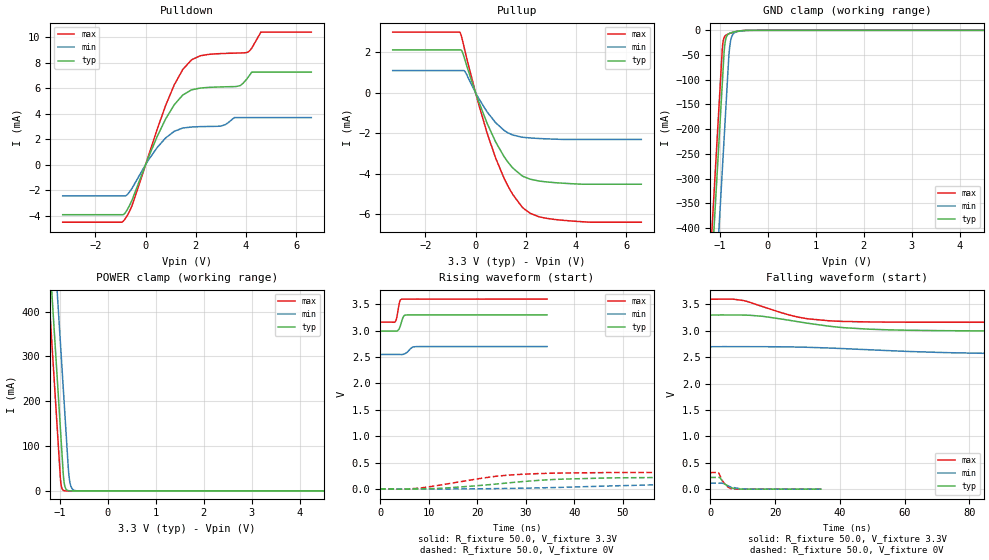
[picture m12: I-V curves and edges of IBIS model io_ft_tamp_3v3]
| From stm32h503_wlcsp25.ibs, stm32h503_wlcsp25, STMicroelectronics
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[Model]   io_ft_tamp_3v3
Model_type I/O
Polarity   Non-Inverting
Enable   Active-Low
| CAP_THRESHOLD on pad IOFT is "UDTCAPC" :
| Rising=20.0% of vddios   Falling=80.0% of vddios
| C_comp min and max val. don't necessarily correlate with the min and max pvt
| but are the smallest and greatest pad capacitance found.
| var   typ   min   max
C_comp   2.63002pF  2.62265pF  2.64550pF
|C_comp_pullup   1.52890pF  1.47780pF  1.43435pF
|C_comp_pulldown   1.10112pF  1.14485pF  1.21115pF
Vinl = 810.0mV
Vinh = 2.52V
Vmeas = 1.65V   | Reference voltage for timing measurements
Cref  = 50.0pF   | Timing specification test load capacitance value
Rref  = 100.0MOhm   | Timing specification test load resistance value
Vref  = 1.65V   | Timing specification test load voltage
[Model Spec]
| TIME_THRESHOLD on pin ZIV11 is "CMOS" :
| Rising=40.0% of vdd   Falling=60.0% of vdd
Vinl 1.29880V 1.07480V 1.40680V
Vinh 1.77520V 1.49320V 1.89720V
| variable   typ   min   max
[Temperature Range] 25.0 125.0 -40.0
| variable   typ   min   max
[Voltage Range] 3.3V 2.7V 3.6V
| variable   typ   min   max
[POWER Clamp Reference] 3.3V 2.7V 3.6V
| variable   typ   min   max
[GND Clamp Reference] 0V 0V 0V
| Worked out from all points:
|   slope of the pulldown table from 0 to 0.495 V, typ, clamps not added: 211 ohm
|   slope of the pullup table from 0 to 0.495 V, typ, clamps not added: 307 ohm
|   GND clamp passes 1 mA (typ) near -0.57 V on its own axis
|   POWER clamp passes 1 mA (typ) near -0.84 V on its own axis
|   rising waveform, R_fixture 50.0, V_fixture 3.3V: 20-80 % time 642ps typ, 1.02ns min, 501ps max; typ from 2.99 V to 3.3 V
|   falling waveform, R_fixture 50.0, V_fixture 3.3V: 20-80 % time 22.1ns typ, 40.9ns min, 14.5ns max; typ from 3.3 V to 2.99 V
|   rising waveform, R_fixture 50.0, V_fixture 0V: 20-80 % time 17.9ns typ, 30.6ns min, 13.4ns max; typ from 0 V to 0.222 V
|   falling waveform, R_fixture 50.0, V_fixture 0V: 20-80 % time 2.43ns typ, 3.42ns min, 2.02ns max; typ from 0.222 V to 0 V
[POWER Clamp]
-3.3V     4.068A     4.259A     3.957A
-1.24V    565.8mA    757.2mA    454.5mA
-1.17V    446.8mA    638.2mA    335.5mA
-1.13V    378.8mA    570.2mA    267.5mA
-1.05V    242.8mA    434.2mA    131.5mA
-980mV    123.8mA    315.2mA    17.95mA
-920mV    26.3mA     213.2mA    906uA
-880mV    5.543mA    145.2mA    123.7uA
-810mV    363.5uA    33.6mA     3.797uA
-770mV    76.62uA    10.47mA    518.9nA
-690mV    3.404uA    1.017mA    9.9nA
6.6V      0A         0A         0A
[GND Clamp]
-3.3V     -4.103A    -4.279A    -4.033A
-1.25V    -618.3mA   -794.4mA   -547.9mA
-960mV    -125.3mA   -301.4mA   -54.9mA
-950mV    -108.3mA   -284.4mA   -38.2mA
-930mV    -74.28mA   -250.4mA   -21.25mA
-910mV    -41.9mA    -216.3mA   -14.37mA
-890mV    -23.93mA   -182.3mA   -11.25mA
-810mV    -6.829mA   -48.78mA   -6.737mA
-780mV    -5.411mA   -23.28mA   -5.701mA
-690mV    -2.92mA    -4.615mA   -3.19mA
-410mV    -72.95uA   -208.4uA   -32.16uA
6.6V      3.146nA    586.1nA    192.6pA
| variable   typ   min   max
[Pullup Reference] 3.3V 2.7V 3.6V
| variable   typ   min   max
[Pulldown Reference] 0V 0V 0V
[Pullup]
-3.3V     2.118mA    1.099mA    3.002mA
-620mV    2.118mA    1.099mA    2.981mA
-540mV    2.047mA    1.099mA    2.683mA
-420mV    1.614mA    1.045mA    2.057mA
120mV     -423.9uA   -273uA     -554.9uA
460mV     -1.518mA   -952.3uA   -2.004mA
800mV     -2.438mA   -1.486mA   -3.239mA
1.29V     -3.439mA   -1.987mA   -4.622mA
1.92V     -4.158mA   -2.21mA    -5.737mA
2.51V     -4.367mA   -2.265mA   -6.134mA
3.19V     -4.454mA   -2.3mA     -6.279mA
6.6V      -4.528mA   -2.313mA   -6.409mA
[Pulldown]
-3.3V     -3.931mA   -2.458mA   -4.52mA
-860mV    -3.894mA   -2.458mA   -4.374mA
-520mV    -2.688mA   -1.793mA   -3.111mA
800mV     3.6mA      2.103mA    4.66mA
1.48V     5.472mA    2.879mA    7.48mA
1.83V     5.88mA     2.962mA    8.24mA
2.99V     6.111mA    3.029mA    8.73mA
3.6V      6.141mA    3.701mA    8.772mA
4.05V     6.784mA    3.701mA    8.828mA
4.23V     7.274mA    3.701mA    9.167mA
4.59V     7.274mA    3.701mA    10.42mA
6.6V      7.274mA    3.701mA    10.42mA
[Ramp]
dV/dt_r 133.32371mV/17.75827ns 68.10059mV/30.01872ns 188.78366mV/13.44463ns
dV/dt_f 183.37683mV/21.75902ns 90.19237mV/40.12235ns 262.38588mV/14.4263ns
R_load = 50.0
| Removed startup time: 0s 0s 0s  .
| Removed end time: 34.4ns.
[Rising Waveform]
R_fixture   = 50.0
V_fixture   = 3.3V
V_fixture_min = 2.7V
V_fixture_max = 3.6V
0s        2.994V     2.55V      3.163V
3.05ns    2.994V     2.55V      3.168V
3.4ns     2.994V     2.55V      3.249V
4ns       3.057V     2.55V      3.55V
4.45ns    3.188V     2.549V     3.597V
4.75ns    3.263V     2.553V     3.599V
5.05ns    3.293V     2.564V     3.599V
6.5ns     3.3V       2.679V     3.599V
7.05ns    3.3V       2.696V     3.6V
34.4ns    3.3V       2.7V       3.6V
| Removed startup time: 0s 0s 0s  .
| Removed end time: 599.4ns.
[Falling Waveform]
R_fixture   = 50.0
V_fixture   = 3.3V
V_fixture_min = 2.7V
V_fixture_max = 3.6V
0s        3.3V       2.7V       3.6V
10.15ns   3.299V     2.7V       3.575V
16.3ns    3.275V     2.7V       3.456V
23.9ns    3.205V     2.696V     3.309V
30.2ns    3.143V     2.688V     3.227V
39.15ns   3.071V     2.669V     3.183V
48.95ns   3.032V     2.642V     3.169V
85.65ns   2.999V     2.573V     3.163V
134.6ns   2.995V     2.555V     3.163V
599.4ns   2.994V     2.55V      3.163V
| Removed startup time: 0s 0s 0s  .
| Removed end time: 599.4ns.
[Rising Waveform]
R_fixture   = 50.0
V_fixture   = 0V
V_fixture_min = 0V
V_fixture_max = 0V
0s        67.41nV    382.4nV    77.77nV
4.2ns     -2.094mV   -30.79uV   -2.95mV
8.1ns     1.219mV    -286.8uV   16.16mV
21.2ns    71.93mV    4.878mV    208.3mV
27ns      121mV      11.8mV     266.8mV
35.6ns    179.6mV    27.28mV    299.9mV
46.9ns    209.6mV    56.18mV    311.4mV
73.4ns    221.4mV    101.4mV    314.5mV
110.1ns   222.1mV    112.3mV    314.6mV
599.4ns   222.2mV    113.5mV    314.6mV
| Removed startup time: 0s 0s 0s  .
| Removed end time: 34.4ns.
[Falling Waveform]
R_fixture   = 50.0
V_fixture   = 0V
V_fixture_min = 0V
V_fixture_max = 0V
0s        222.2mV    113.5mV    314.6mV
2.5ns     222mV      113.5mV    314.3mV
3ns       216.3mV    113.5mV    255.8mV
3.65ns    162.5mV    114.5mV    167.2mV
4.45ns    99.12mV    93.46mV    102.5mV
5.7ns     51.26mV    56.88mV    31.54mV
6.75ns    22.28mV    35.05mV    4.945mV
8.45ns    2.15mV     17.65mV    594.4uV
11.95ns   275.1uV    1.242mV    207.9uV
34.4ns    50.41uV    45.43uV    48.34uV
